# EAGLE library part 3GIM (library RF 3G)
3GIM This is a kind of 3G RF modeule. http://tabrain.jp/data/3GIM_Manual_V01R01.pdf
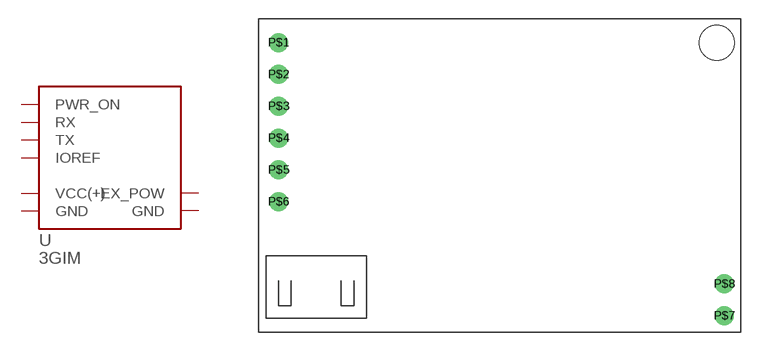
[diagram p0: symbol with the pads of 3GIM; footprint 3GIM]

Designator prefix U

## 3GIM  [3GIM]
P$1  PWR_ON  in
P$2  RX  in
P$3  TX  out
P$4  IOREF  in
P$5  VCC(+)  pwr
P$6  GND  pwr
P$7  GND  pwr
P$8  EX_POW  pwr

## Footprint 3GIM (pad centres in mm)
3GIM This is a kind of 3G RF modeule. http://tabrain.jp/data/3GIM_Manual_V01R01.pdf
drill 1: P$1 -35,0; P$2 -35,-2.54; P$3 -35,-5.08; P$4 -35,-7.62; P$5 -35,-10.16; P$6 -35,-12.7; P$7 0.6,-21.8; P$8 0.6,-19.26
hole 2.8 at 0,0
